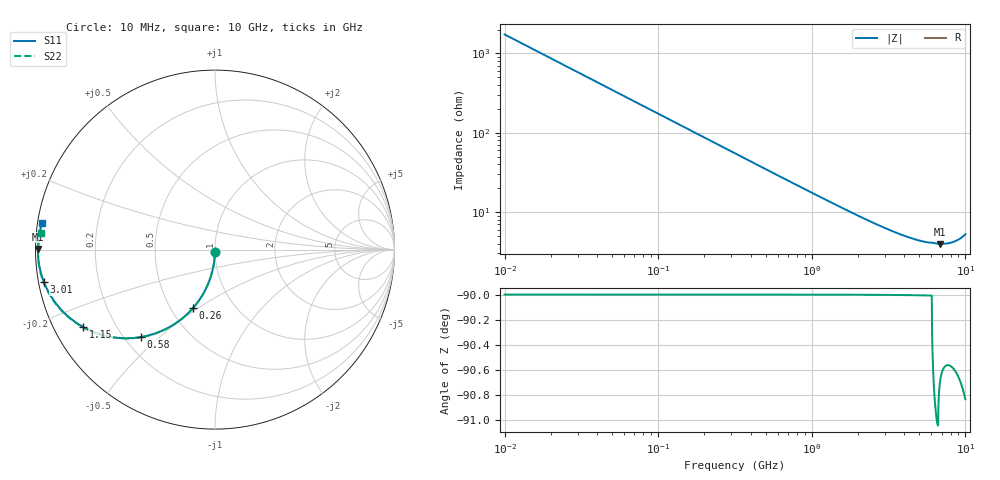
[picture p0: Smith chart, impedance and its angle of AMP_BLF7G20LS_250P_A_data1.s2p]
! Created Thu Oct 28 10:30:08 2010
# ghz S ma R 50
! 2 Port Network Data from SP1.SP block
! freq  magS11  angS11  magS21  angS21  magS12  angS12  magS22  angS22
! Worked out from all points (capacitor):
!   1000 points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, 10 MHz to 10 GHz, reference 50 ohm
!   read as one part in shunt: C = 9.18 pF near 60 MHz
!   lowest |Z| = 3.95 ohm at 6.85 GHz (marker M1)
!   S11 on the Smith chart (normalised r, x): 10 MHz: 1.00, -0.03; 260 MHz: 0.64, -0.48; 580 MHz: 0.27, -0.44; 1.15 GHz: 0.09, -0.27; 3.01 GHz: 0.02, -0.09; 10 GHz: 0.01, +0.08
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0.01  0.01435 -90.8  0.9999 -0.8  0.9999 -0.8  0.01435 -90.8
0.04  0.05729 -93.3  0.9984 -3.3  0.9984 -3.3  0.05729 -93.3
0.07  0.09992 -95.8  0.995 -5.8  0.995 -5.8  0.09992 -95.8
0.09  0.1281 -97.4  0.9918 -7.4  0.9918 -7.4  0.1281 -97.4
0.11  0.1559 -99.1  0.9878 -9.1  0.9878 -9.1  0.1559 -99.1
0.14  0.1969 -101.5  0.9804 -11.5  0.9804 -11.5  0.1969 -101.5
0.17  0.2369 -103.9  0.9715 -13.9  0.9715 -13.9  0.2369 -103.8
0.26  0.3493 -110.7  0.937 -20.7  0.937 -20.7  0.3493 -110.7
0.4  0.4971 -120.2  0.8677 -30.2  0.8677 -30.2  0.4971 -120.1
0.58  0.6384 -130.3  0.7697 -40.2  0.7697 -40.2  0.6384 -130.1
0.85  0.7711 -141.3  0.6367 -51.2  0.6367 -51.2  0.7711 -141.1
1.15  0.8523 -149.6  0.523 -59.5  0.523 -59.5  0.8523 -149.4
1.39  0.8906 -154.4  0.4547 -64.2  0.4547 -64.2  0.8906 -154.1
1.68  0.92 -158.7  0.3918 -68.5  0.3918 -68.5  0.92 -158.3
2.24  0.9508 -164.3  0.3097 -74.1  0.3097 -74.1  0.9508 -163.8
3.01  0.9698 -169.2  0.2438 -78.8  0.2438 -78.8  0.9698 -168.5
3.34  0.9743 -170.7  0.225 -80.3  0.225 -80.3  0.9743 -169.9
5.01  0.9849 -176.1  0.173 -85.5  0.173 -85.5  0.9849 -174.9
6.67  0.9846 -179.8  0.1569 -89.9  0.1569 -89.9  0.9855 -178.1
6.85  0.9853 179.8  0.1569 -90.0  0.1569 -90.0  0.986 -178.5
8.34  0.9841 176.4  0.166 -93.0  0.166 -93.0  0.9847 178.7
10  0.975 171.3  0.2061 -97.9  0.2061 -97.9  0.976 174.7
